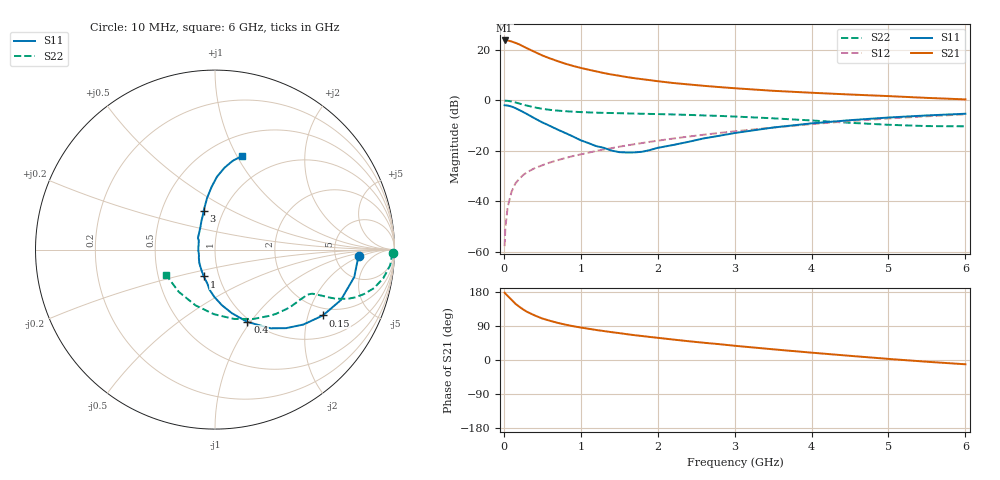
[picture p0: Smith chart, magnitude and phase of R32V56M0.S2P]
! SIEMENS Small Signal Semiconductors
! BFR181
! Si NPN RF Bipolar Junction Transistor in SOT23
! VCE = 2.5 V  IC = 6 mA
! Common Emitter S-Parameters:  May  1996
# GHz  S  MA  R  50
!  f  S11  S21  S12  S22
! GHz  MAG  ANG  MAG  ANG  MAG  ANG  MAG  ANG
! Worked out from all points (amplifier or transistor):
!   36 points, 10 MHz to 6 GHz, reference 50 ohm
!   highest |S21| = 23.7 dB at 10 MHz (marker M1)
!   |S21| within 3 dB of that: start of sweep to 294.5 MHz
!   unconditionally stable (mu >= 1): 974.8 MHz to 2.855 GHz
!   at 250 MHz: K = 0.48, MSG = 25.5 dB, |S12| = -29.6 dB
!   at 1.4 GHz: K = 1.06, MAG = 13.1 dB, |S12| = -18.9 dB
!   at 6 GHz: K = 0.86, MSG = 3.0 dB, |S12| = -5.5 dB
!   S11 on the Smith chart (normalised r, x): 10 MHz: 8.82, -1.67; 150 MHz: 1.72, -2.50; 400 MHz: 0.96, -0.97; 1 GHz: 0.85, -0.26; 3 GHz: 0.81, +0.37; 6 GHz: 0.71, +1.05
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0.01  0.8027 -2.4  15.37 177.7  0.0013 92.0  0.9901 -1.0
0.02  0.7966 -4.4  15.25 175.3  0.003 82.4  0.9859 -2.0
0.05  0.791 -11.1  15.34 169.2  0.0078 84.2  0.98 -5.1
0.1  0.7553 -21.9  14.67 159.1  0.0155 79.6  0.9513 -9.6
0.15  0.7043 -31.4  13.8 148.6  0.0227 73.7  0.9119 -13.6
0.2  0.6455 -40.3  12.86 140.7  0.028 70.8  0.8665 -16.6
0.25  0.5906 -47.8  11.76 133.6  0.0332 67.9  0.8258 -18.8
0.3  0.5373 -54.7  10.78 127.3  0.0377 66.9  0.7896 -20.3
0.4  0.4417 -65.9  9.141 117.7  0.0454 65.2  0.7278 -22.1
0.5  0.3667 -75.1  7.759 109.5  0.052 64.6  0.6809 -22.9
0.6  0.3123 -82.9  6.772 103.5  0.059 64.4  0.6502 -23.3
0.7  0.2637 -90.8  5.989 98.0  0.0655 64.6  0.6278 -23.7
0.8  0.2261 -97.7  5.325 93.3  0.0723 64.8  0.6109 -24.0
1  0.1623 -112.7  4.398 85.7  0.0854 65.7  0.5868 -24.9
1.1  0.1428 -120.5  4.053 82.5  0.0923 65.9  0.5789 -25.5
1.6  0.093 -176.7  2.896 68.1  0.1283 65.6  0.5532 -29.9
2.2  0.1309 131.9  2.212 54.0  0.1756 63.7  0.5273 -37.3
3  0.2257 106.2  1.741 37.6  0.2439 58.4  0.4794 -50.2
3.5  0.2903 98.8  1.549 28.2  0.2903 54.2  0.4418 -61.0
4.5  0.4055 88.5  1.308 11.0  0.3897 43.7  0.3601 -90.9
5.5  0.5038 78.8  1.121 -4.6  0.4851 30.9  0.3101 -130.5
6  0.5442 73.8  1.047 -11.3  0.5291 23.8  0.3066 -152.3
